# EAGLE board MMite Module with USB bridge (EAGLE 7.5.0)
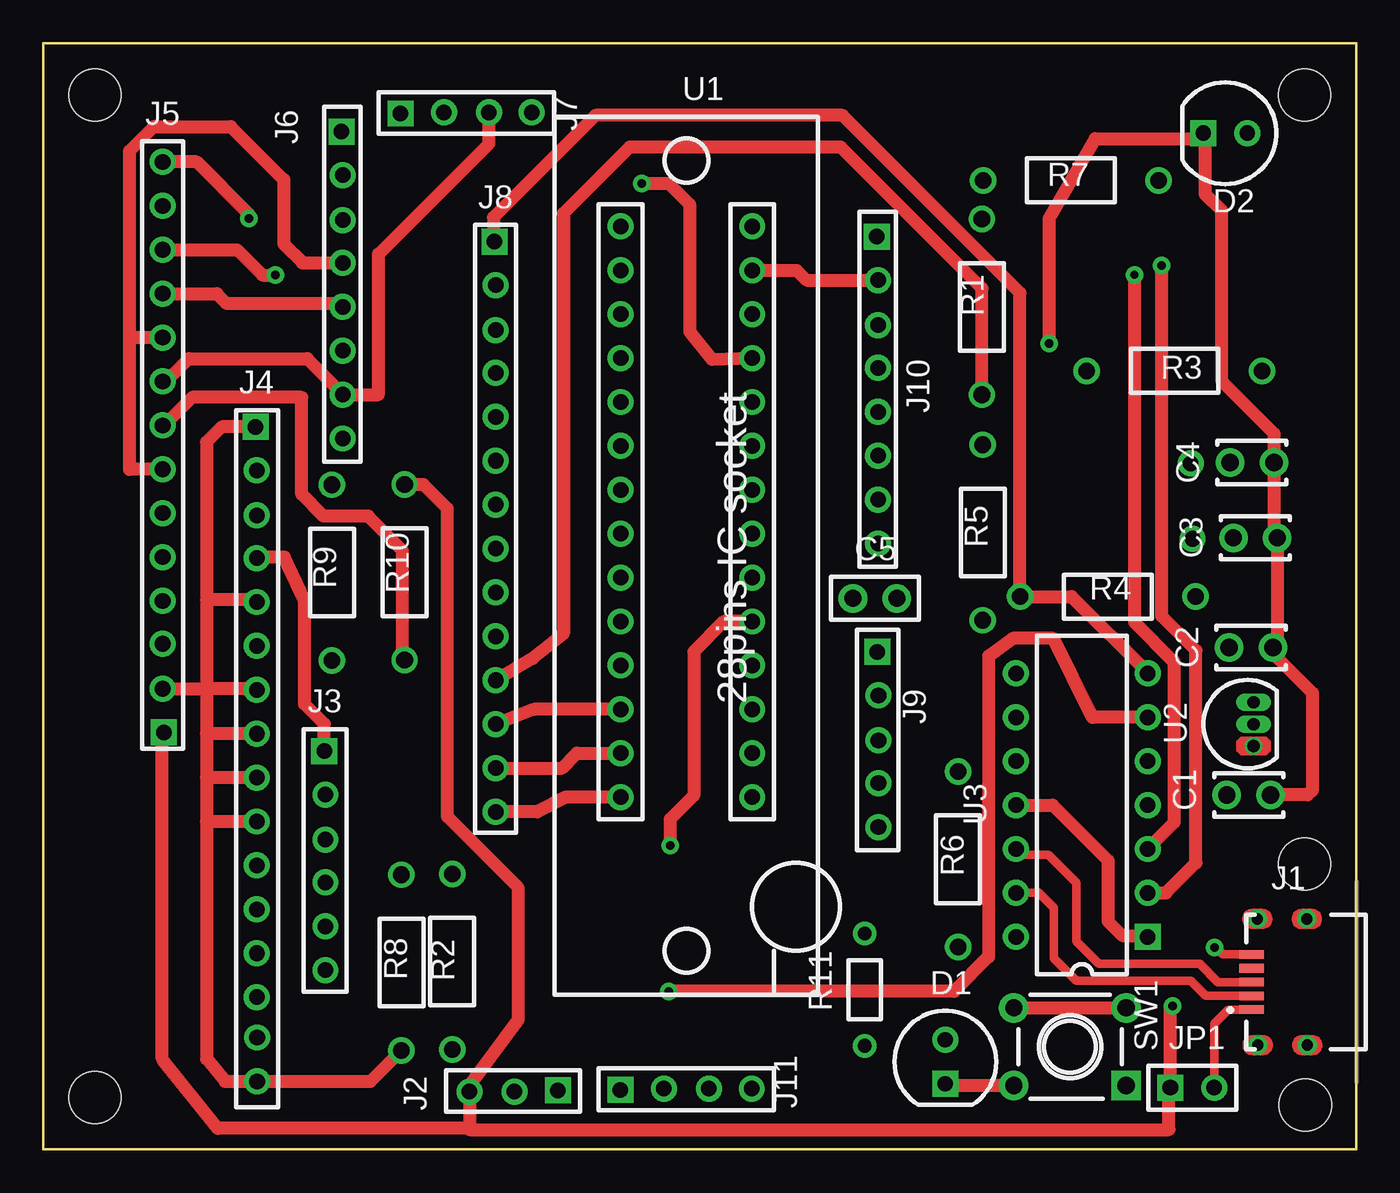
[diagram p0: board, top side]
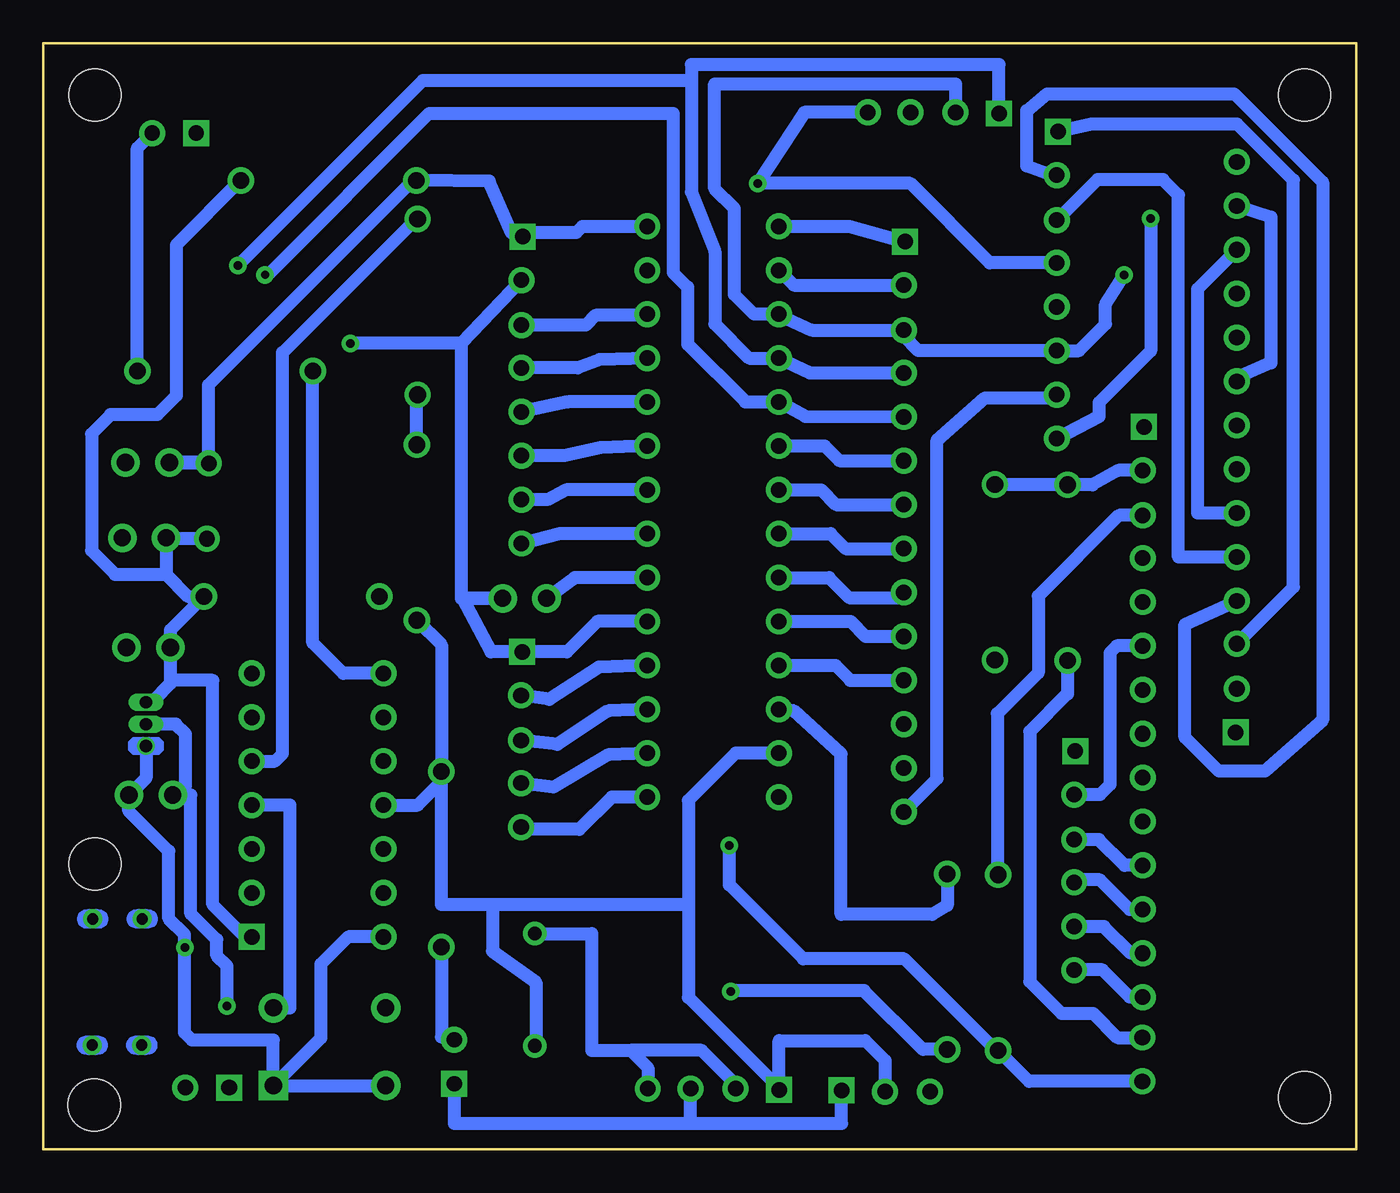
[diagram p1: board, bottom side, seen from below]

Size 76 x 64 mm. Coordinates in mm from the lower left corner, seen from the top.
Outline: 0,64 76,64 76,0 0,0 0,64
Copper layers (1*16): Top 0.035mm / dielectric 1.5mm / Bottom 0.035mm
Design rules "default *": minimum track width 10mil, minimum drill 0.61mm, track to track 8mil, track to pad 8mil, pad to pad 8mil, via to via 8mil, smd to smd 8mil, copper to edge 40mil, drill to drill 8mil, minimum pad ring 0mil, minimum via ring 8mil, stop-mask expansion 4mil, vias tented up to drill 19mil, thermal gap 10mil
Net classes: 0 Default: width 0.5 mm, clearance 0.33 mm
Holes 3 mm at 73.05,2.58 3,3 3,61 73,61 73,16.5

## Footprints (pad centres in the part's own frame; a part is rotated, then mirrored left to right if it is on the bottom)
CAP-2.54/4x2.5 = drill 1 pad 1.65: 1 -1.27,0; 2 1.27,0
CAP-2.54/5.1x2.5 = drill 1 pad 1.65: 1 -1.27,0; 2 1.27,0
LED-5Cil_Red = drill 0.889 pad 1.5 square: 1 -1.27,0 | drill 0.889 pad 1.5: 2 1.27,0
LED-5Cil_Green = drill 0.889 pad 1.5 square: 1 -1.27,0 | drill 0.889 pad 1.5: 2 1.27,0
Mini_USB_51387-578 = smd 0.5 x 1.4: 1 -1.6,1.75; 2 -0.8,1.75; 3 0,1.75; 4 0.8,1.75; 5 1.6,1.75 | drill 0.65 pad 1.1: 6 -3.65,1.396; 7 3.648,1.421; 8 -3.65,-1.472; 9 3.647,-1.447
CON3F = drill 0.9 pad 1.5 square: 1 -0.033,2.561 | drill 0.9 pad 1.5: 2 0.033,0.043; 3 0.033,-2.561
CON6F = drill 0.9 pad 1.5 square: 1 -0.033,6.339 | drill 0.9 pad 1.5: 2 0.033,3.821; 3 0.033,1.217; 4 0.033,-1.259; 5 0.033,-3.799; 6 0.033,-6.339
CON16F = drill 0.9 pad 1.5 square: 1 -0.044,18.937 | drill 0.9 pad 1.5: 2 0.022,16.419; 3 0.022,13.815; 4 0.022,11.339; 5 0.022,8.799; 6 0.022,6.259; 7 0.022,3.719; 8 0.022,1.179; 9 0.022,-1.361; 10 0.022,-3.901; 11 0.022,-6.441; 12 0.022,-8.981; 13 0.022,-11.521; 14 0.022,-14.061; 15 0.044,-16.397; 16 0.044,-18.937
CON14F = drill 0.9 pad 1.5 square: 1 -0.033,16.499 | drill 0.9 pad 1.5: 2 0.033,13.981; 3 0.033,11.377; 4 0.033,8.901; 5 0.033,6.361; 6 0.033,3.821; 7 0.033,1.281; 8 0.033,-1.259; 9 0.033,-3.799; 10 0.033,-6.339; 11 0.033,-8.879; 12 0.033,-11.419; 13 0.033,-13.959; 14 0.033,-16.499
CON8F = drill 0.9 pad 1.5 square: 1 -0.033,8.879 | drill 0.9 pad 1.5: 2 0.033,6.361; 3 0.033,3.757; 4 0.033,1.281; 5 0.033,-1.259; 6 0.033,-3.799; 7 0.033,-6.339; 8 0.033,-8.879
CON4F = drill 0.9 pad 1.5 square: 1 -0.033,3.799 | drill 0.9 pad 1.5: 2 0.033,1.281; 3 0.033,-1.323; 4 0.033,-3.799
CON5F = drill 0.9 pad 1.5 square: 1 -0.033,5.069 | drill 0.9 pad 1.5: 2 0.033,2.551; 3 0.033,-0.053; 4 0.033,-2.529; 5 0.033,-5.069
HDR-1x2 = drill 0.9 pad 1.5 square: 1 -1.27,0 | drill 0.9 pad 1.5: 2 1.27,0
Pad = drill 0.9 pad 1.5: 1 0,0
RES-10.16/5.1x2.5 = drill 0.965 pad 1.524: 1 -5.08,0; 2 5.08,0
RES-10.16/5.1x2.5_R3 = drill 0.965 pad 1.524: 1 -5.08,0; 2 5.08,0
RES-6.5/3.4x1.9 = drill 0.8 pad 1.35: 1 -3.25,0; 2 3.25,0
B3F-1 = drill 1 pad 1.7 square: 1 -3.25,2.25 | drill 1 pad 1.7: 2 3.25,2.25; 3 -3.25,-2.25; 4 3.25,-2.25
28pins_ZIF_pattern = drill 0.9 pad 1.5: 1 -3.81,17.78; 2 -3.81,15.24; 3 -3.81,12.7; 4 -3.81,10.16; 5 -3.81,7.62; 6 -3.81,5.08; 7 -3.81,2.54; 8 -3.81,0; 9 -3.81,-2.54; 10 -3.81,-5.08; 11 -3.81,-7.62; 12 -3.81,-10.16; 13 -3.81,-12.7; 14 -3.81,-15.24; 15 3.81,-15.24; 16 3.81,-12.7; 17 3.81,-10.16; 18 3.81,-7.62; 19 3.81,-5.08; 20 3.81,-2.54; 21 3.81,0; 22 3.81,2.54; 23 3.81,5.08; 24 3.81,7.62; 25 3.81,10.16; 26 3.81,12.7; 27 3.81,15.24; 28 3.81,17.78
TO-92 = drill 0.7 pad 1: 1 -1.27,0 | drill 0.7 pad 1 long: 2 0,0; 3 1.27,0
DIP-14 = drill 0.9 pad 1.5 square: 1 -3.81,7.62 | drill 0.9 pad 1.5: 2 -3.81,5.08; 3 -3.81,2.54; 4 -3.81,0; 5 -3.81,-2.54; 6 -3.81,-5.08; 7 -3.81,-7.62; 8 3.81,-7.62; 9 3.81,-5.08; 10 3.81,-2.54; 11 3.81,0; 12 3.81,2.54; 13 3.81,5.08; 14 3.81,7.62

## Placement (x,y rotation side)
C1  10uF  [CAP-2.54/4x2.5]  69.77,20.51 0 top
C2  10uF  [CAP-2.54/4x2.5]  69.91,29.04 0 top
C3  100nF  [CAP-2.54/4x2.5]  70.15,35.39 0 top
C4  100nF  [CAP-2.54/4x2.5]  69.96,39.74 0 top
C5  47uF-16V Tan  [CAP-2.54/5.1x2.5]  48.14,31.88 0 top
D1  RED  [LED-5Cil_Red]  52.21,5.07 90 top
D2  GREEN  [LED-5Cil_Green]  68.42,58.79 0 top
J1  MINI USB  [Mini_USB_51387-578]  71.69,9.68 90 top
J2  POWER I/O  [CON3F]  27.23,3.38 270 top
J3  LCD 16X2  [CON6F]  16.3,16.71 0 top
J4  CON16F  [CON16F]  12.34,22.87 0 top
J5  CON14F  [CON14F]  6.95,40.63 180 top
J6  LCD ILI9341  [CON8F]  17.3,50.01 0 top
J7  ILI9341-SD  [CON4F]  24.48,59.96 90 top
J8  MM I/O  [CON14F]  26.15,36.02 0 top
J9  MM I/O  [CON5F]  48.31,23.71 0 top
J10  MM I/O  [CON8F]  48.28,43.93 0 top
J11  UNI/O-TEMP  [CON4F]  37.21,3.48 90 top
JP1  JUMPER  [HDR-1x2]  66.51,3.58 0 top
Pad1  PAD  [Pad]  66.41,39.69 0 top
Pad2  PAD  [Pad]  66.53,35.33 0 top
R1  1K5  [RES-10.16/5.1x2.5]  54.33,48.74 270 top
R2  1K5  [RES-10.16/5.1x2.5]  23.67,10.86 90 top
R3  1K  [RES-10.16/5.1x2.5_R3]  65.47,45.04 0 top
R4  10K  [RES-10.16/5.1x2.5_R3]  61.62,31.98 180 top
R5  10K  [RES-10.16/5.1x2.5]  54.38,35.69 90 top
R6  1K5  [RES-10.16/5.1x2.5]  52.95,16.78 270 top
R7  10R  [RES-10.16/5.1x2.5_R3]  59.48,56.06 180 top
R8  1K8  [RES-10.16/5.1x2.5]  20.74,10.81 270 top
R9  1K8  [RES-10.16/5.1x2.5]  16.71,33.37 270 top
R10  18R  [RES-10.16/5.1x2.5]  20.92,33.39 270 top
R11  100K  [RES-6.5/3.4x1.9]  47.55,9.24 90 top
SW1  SWITCH_2DIP  [B3F-1]  59.43,5.94 180 top
U1  28PINS_ZIF_SOCKET  [28pins_ZIF_pattern]  37.23,35.62 0 top
U2  MCP1700-33  [TO-92]  70.05,24.61 90 top
U3  PIC16F1455  [DIP-14]  60.11,19.92 180 top

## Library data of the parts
C1-C4 = common; DESCRIPTION: Non-polarized
C5 = common; ATTR_1: Electrolytic; DESCRIPTION: Polarized
D1 D2 = common; DESCRIPTION: LED
J1 J2 J7 J11 = common; DATASHEET: http://datasheets.diptrace.com/con_board_in/510221400_sd.pdf; MANUFACTURER: Molex
J3 J5 J8-J10 JP1 Pad1 Pad2 = common
J4 = common; DATASHEET: http://datasheets.diptrace.com/con_board_in/DF4.pdf; MANUFACTURER: Hirose
J6 = common; DATASHEET: http://datasheets.diptrace.com/con_board_in/510150300_sd.pdf; MANUFACTURER: Molex
R1-R11 = common; DESCRIPTION: Fixed Resistor
SW1 = common; ATTR_1: 2 Positions; DESCRIPTION: DIP Switch
U1 = common; MANUFACTURER: MICROMITE
U2 = common; DATASHEET: http://datasheets.diptrace.com/microchip/22008d.pdf; MANUFACTURER: Microchip
U3 = common; DATASHEET: http://datasheets.diptrace.com/microchip/21203Q.pdf; MANUFACTURER: Microchip

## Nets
Net_0: J8.1 R4.2 U1.1 U3.7
Net_1: C1.2 C2.2 C3.2 C4.2 C5.2 D1.1 D2.1 J1.5 J2.1 J4.1 J4.5 J4.7 J4.8 J4.9 J4.10 J4.16 J5.2 J9.1 J10.2 J11.3 R8.2 SW1.1 SW1.2 U1.19 U1.27 U2.1 U3.14
Net_2: C2.1 C3.1 J2.2 J8.13 J11.1 Pad2.1 R4.1 R5.1 R6.1 R7.1 R11.1 U1.13 U2.3 U3.1 U3.11
Net_3: J7.1 J8.4 U1.4 U3.2
Net_4: J8.5 U1.5 U3.3
Net_5: SW1.3 SW1.4 U3.4
Net_6: R1.1 U3.5
Net_7: J8.11 R1.2 R5.2 U1.11
Net_8: R2.1 U3.6
Net_9: J8.12 R2.2 U1.12
Net_10: R3.1 U3.8
Net_11: J1.3 U3.12
Net_12: D2.2 R3.2
Net_13: J1.2 U3.13
Net_14: C1.1 J1.1 J2.3 J4.2 J5.1 JP1.1 JP1.2 R9.1 R10.1 U2.2
Net_15: C5.1 U1.20
Net_16: D1.2 R6.2
Net_17: C4.1 J10.1 Pad1.1 R7.2 U1.28
Net_18: J3.1 J4.4
Net_19: J4.3 R8.1
Net_20: J11.2 J11.4 R11.2
Net_21: J3.6 J4.14
Net_22: J3.5 J4.13
Net_23: J3.4 J4.12
Net_24: J3.3 J4.11
Net_25: J3.2 J4.6
Net_26: J4.15 R9.2
Net_27: J9.2 U1.18
Net_28: J9.3 U1.17
Net_29: J9.4 U1.16
Net_30: J9.5 U1.15
Net_31: J10.3 U1.26
Net_32: J5.7 J5.10 J6.4 J7.4 J10.4 U1.25
Net_33: J10.5 U1.24
Net_34: J10.6 U1.23
Net_35: J10.7 U1.22
Net_36: J10.8 U1.21
Net_37: J8.2 U1.2
Net_38: J5.6 J5.12 J6.6 J7.2 J8.3 U1.3
Net_39: J8.6 U1.6
Net_40: J8.7 U1.7
Net_41: J8.8 U1.8
Net_42: J8.9 U1.9
Net_43: J8.10 U1.10
Net_44: J5.9 J5.13 J6.7 J7.3 J8.14 U1.14
Net_45: J5.8 R10.2
Net_49: J5.14 J6.8
Net_50: J5.11 J6.5
Net_51: J5.5 J6.3
Net_52: J5.4 J6.2
Net_53: J5.3 J6.1

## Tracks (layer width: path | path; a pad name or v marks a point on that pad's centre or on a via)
Net_0
  Top 0.75: J8.1 26.06,52.42 26.06,53.92 31.97,59.83 46.26,59.83 56.54,49.55 R4.2 59.52,31.98 63.92,27.58 U3.7
  Bottom 0.75: U1.1 29.33,53.4 J8.1
Net_1  (via drill 0.49 pad 1.02)
  Top 0.5: J1.5 68.28,11.28 67.89,11.67 v67.79,11.67
  Top 0.75: SW1.2 52.21,3.69 D1.1 | v58.22,46.64 58.22,53.87 60.89,58.48 66.83,58.48 D2.1 67.24,58.8 67.24,55.27 68.19,54.33 68.19,44.47 71.23,41.43 C4.2 71.23,35.58 C3.2 71.42,29.28 C2.2 71.18,28.69 73.45,26.42 73.45,20.79 73.17,20.51 C1.2 | U1.27 43.61,50.86 44.18,50.29 J10.2 | U1.19 39.41,30.54 37.65,28.79 37.65,20.48 36.28,19.11 v36.28,17.57 | J4.1 10.33,41.81 9.46,40.93 9.46,31.8 | 9.46,31.8 9.46,26.65 | 9.46,26.65 9.46,24.05 | 9.46,24.05 9.46,21.51 | 9.46,21.51 9.46,18.97 | 9.46,18.97 9.46,5.23 10.53,3.93 J4.16 18.94,3.93 R8.2 | J4.5 12.36,31.8 9.46,31.8 | J4.7 12.36,26.65 9.46,26.65 | J4.8 9.46,24.05 | J4.9 9.46,21.51 | J4.10 9.46,18.97 | J5.2 9.46,26.65
  Bottom 0.75: SW1.1 SW1.2 | SW1.2 | J10.2 51.8,46.64 | 51.8,46.64 v58.22,46.64 | 51.8,46.64 51.8,31.88 C5.2 51.73,31.88 50.09,28.78 J9.1 45.68,28.78 43.92,30.54 U1.19 | SW1.1 62.68,6.33 67.38,6.33 67.82,6.76 67.82,11.63 | 67.82,11.63 67.82,12.45 68.72,13.35 68.72,17.26 71.04,19.57 C1.2 70.05,21.5 U2.1 | D1.1 52.21,1.5 38.55,1.5 | 38.55,1.5 29.79,1.5 J2.1 | J11.3 38.55,3.51 38.55,1.5 | v67.79,11.67 67.82,11.63 | U3.14 58.35,12.3 59.93,10.72 59.93,6.43 SW1.1 | v36.28,17.57 36.28,15.3 32.01,11.02 26.16,11.02 20.86,5.73 R8.2 18.94,3.93 J4.16
Net_2
  Top 0.75: J8.13 30.02,22.06 30.88,22.92 U1.13 | U3.11 58.43,19.92 61.63,16.72 61.63,13.2 62.47,12.37 63.86,12.37 U3.1
  Bottom 0.75: 68.88,33.27 C3.1 68.83,35.33 Pad2.1 | 68.88,33.27 67.6,31.98 R4.1 68.64,30.04 C2.1 68.64,26.94 69.7,25.88 | R5.1 52.95,29.19 R6.1 | R7.1 68.3,52.32 68.3,43.6 69.39,42.51 72.1,42.51 73.2,41.4 73.2,34.64 71.83,33.27 68.88,33.27 | J2.2 27.27,5.15 28.41,6.3 33.41,6.3 J11.1 33.41,3.56 38.65,8.8 38.65,14.16 | U1.13 35.92,22.92 38.65,20.19 38.65,14.16 | 38.65,14.16 49.99,14.16 | 49.99,14.16 49.99,11.47 47.48,9.66 47.48,5.99 R11.1 | U3.1 64.33,12.3 66.19,14.16 66.19,27.13 68.45,27.13 69.7,25.88 | 69.7,25.88 U2.3 69.7,25.88 | 49.99,14.16 52.95,14.16 R6.1 | U3.11 54.32,19.92 52.95,21.29 R6.1
Net_3  (via drill 0.49 pad 1.02)
  Top 0.75: U3.2 64.98,14.84 66.72,16.58 66.72,28.88 64.74,30.85 v64.74,51.13
  Bottom 0.75: J8.4 31.62,44.92 U1.4 35.15,45.78 37.12,47.76 37.12,51.95 38.48,55.38 38.48,61.86 | J7.1 20.68,62.76 38.48,62.76 38.48,61.86 | v64.74,51.13 54.02,61.86 38.48,61.86
Net_4  (via drill 0.49 pad 1.02)
  Top 0.75: v63.16,50.6 63.16,30.52 65.45,28.23 65.45,18.9 U3.3
  Bottom 0.75: J8.5 31.89,42.41 U1.5 35.37,43.24 38.7,46.58 38.7,49.88 39.54,50.72 39.54,59.95 53.66,59.95 63.11,50.49 v63.16,50.6
Net_5
  Top 0.75: SW1.4 | SW1.4 SW1.3
  Bottom 0.75: SW1.3 61.72,8.19 61.72,19.92 U3.4
Net_6
  Bottom 0.75: U3.5 62.59,22.46 62.14,22.9 62.14,46.1 54.41,53.82 R1.1
Net_7
  Top 0.75: R1.2 54.33,49.82 46.17,57.98 33.95,57.98 30.11,54.15 30.11,29.84 28.33,28.4 J8.11
  Bottom 0.75: U1.11 30.14,28 29.28,27.14 J8.11 | R5.2 54.38,43.66 R1.2
Net_8  (via drill 0.49 pad 1.02)
  Top 0.75: U3.6 60.73,25 58.46,29.56 56.12,29.56 54.72,28.53 54.72,11.13 52.73,9.14 v36.2,9.14
  Bottom 0.75: R2.1 25.07,5.78 28.48,9.19 36.2,9.19 v36.2,9.14
Net_9
  Top 0.75: U1.12 28.39,25.46 J8.12
  Bottom 0.75: R2.2 23.67,14.12 24.55,13.6 29.82,13.6 29.82,22.88 32.56,25.37 U1.12
Net_10
  Bottom 0.75: U3.8 58.63,27.54 60.39,29.3 R3.1
Net_11
  Top 0.5: J1.3 68,9.68 66.95,10.73 61.11,10.73 59.8,12.03 59.8,15.41 58.16,17.06 56.63,17.06 U3.12
Net_12
  Bottom 0.75: R3.2 70.55,57.93 D2.2
Net_13
  Top 0.5: J1.2 67.3,8.88 66.42,9.77 59.8,9.77 58.5,11.07 58.5,13.97 57.63,14.84 U3.13
Net_14  (via drill 0.49 pad 1.02)
  Top 0.5: JP1.2 67.78,7.27 68.59,8.08 J1.1
  Top 0.75: J2.3 | J2.3 24.67,1.22 | 24.67,1.22 10.1,1.22 6.89,5.23 6.89,23.68 J5.1 | R10.1 21.99,38.48 23.38,37.09 23.38,19.26 27.48,15.16 27.48,7.47 24.56,3.54 J2.3 | v65.36,8.3 65.23,8.17 JP1.1 65.16,3.5 65.16,1.14 24.67,1.14 24.67,1.22 | J2.3
  Bottom 0.75: 20.49,38.45 R10.1 | R10.1 | J4.2 13.79,39.29 15.27,38.45 R9.1 16.81,38.48 R10.1 | U2.2 68.33,24.61 67.76,24.04 67.76,21.02 68.5,20.28 C1.1 67.46,20.51 67.46,13.63 65.95,12.13 65.95,11.21 65.36,10.62 v65.36,8.3
Net_15
  Bottom 0.75: U1.20 45.24,33.08 47.11,31.7 C5.1
Net_16
  Bottom 0.75: R6.2 52.95,6.5 52.21,6.5 D1.2
Net_17
  Bottom 0.75: J10.1 48.67,52.81 48.9,53.05 | 48.9,53.05 50.18,56.03 R7.2 54.4,56.27 66.45,44.22 66.45,39.75 C4.1 68.64,39.69 Pad1.1 | U1.28 44.8,53.39 45.15,53.05 48.9,53.05
Net_18
  Top 0.75: J3.1 16.27,24.62 15.13,25.76 15.13,31.73 13.95,34.27 12.36,34.27 J4.4
Net_19
  Bottom 0.75: J4.3 13.74,36.69 18.41,32.01 18.41,27.57 20.78,25.21 20.78,15.93 R8.1
Net_20
  Bottom 0.75: R11.2 44.26,12.49 44.26,5.73 42.02,5.73 | 42.02,5.73 41.01,4.72 J11.4 | J11.2 35.93,3.76 37.89,5.73 42.02,5.73
Net_21
  Bottom 0.75: J4.14 13.12,8.81 14.7,10.38 16.32,10.38 J3.6
Net_22
  Bottom 0.75: J4.13 13.06,11.35 14.6,12.9 16.32,12.9 J3.5
Net_23
  Bottom 0.75: J4.12 13.12,13.89 14.83,15.6 16.18,15.6 J3.4
Net_24
  Bottom 0.75: J4.11 13.4,16.43 14.89,17.92 J3.3
Net_25
  Bottom 0.75: J4.6 13.86,29.13 14.26,28.73 14.26,21.1 14.84,20.53 J3.2
Net_26
  Bottom 0.75: R9.2 16.71,26.35 18.9,24.17 18.9,9.71 17.06,7.87 15.23,7.87 13.83,6.47 J4.15
Net_27
  Bottom 0.75: U1.18 43.83,27.91 46.7,26.04 J9.2
Net_28
  Bottom 0.75: U1.17 43.3,25.37 46.23,23.43 J9.3
Net_29
  Bottom 0.75: U1.16 43.31,22.83 46.47,20.96 J9.4
Net_30
  Bottom 0.75: U1.15 43.1,20.38 44.97,18.51 48.21,18.51 J9.5
Net_31
  Bottom 0.75: U1.26 41.23,48.25 44.03,48.25 44.59,47.69 J10.3
Net_32  (via drill 0.49 pad 1.02)
  Top 0.75: U1.25 38.73,45.69 37.43,47.31 37.43,54.66 36.21,55.88 v34.65,55.88 | J5.10 5,46.97 | 5,46.97 5,57.77 6.41,59.18 10.86,59.18 13.93,56.11 13.93,52.37 15.01,51.29 J6.4 | J5.7 5,39.35 5,46.97
  Bottom 0.75: U1.25 43.8,45.69 45.05,45.21 J10.4 | J6.4 21.22,51.29 25.82,55.88 v34.65,55.88 31.95,60 J7.4
Net_33
  Bottom 0.75: U1.24 45.64,43.24 J10.5
Net_34
  Bottom 0.75: U1.23 43.75,40.61 45.82,40.13 J10.6
Net_35
  Bottom 0.75: U1.22 45.74,38.16 46.81,37.59 J10.7
Net_36
  Bottom 0.75: U1.21 46.09,35.62 J10.8
Net_37
  Bottom 0.75: U1.2 32.56,50 J8.2
Net_38  (via drill 0.49 pad 1.02)
  Top 0.75: J5.12 11.22,52.05 12.69,50.58 v13.44,50.58
  Bottom 0.75: J7.2 23.2,61.64 37.13,61.64 37.13,55.59 35.99,54.45 35.99,49.46 34.86,48.32 U1.3 33.34,48.25 31.52,47.4 J8.3 26.19,47.03 25.36,46.21 J6.6 16.06,46.21 14.52,47.75 14.52,48.89 13.4,50.66 v13.44,50.58 | J5.6 9.18,36.81 9.18,49.78 J5.12
Net_39
  Bottom 0.75: U1.6 30.77,40.7 29.91,39.84 J8.6
Net_40
  Bottom 0.75: U1.7 30.97,38.16 30.11,37.3 J8.7
Net_41
  Bottom 0.75: U1.8 30.42,35.62 29.56,34.76 J8.8
Net_42
  Bottom 0.75: U1.9 30.52,33.08 29.35,31.92 26.49,31.92 J8.9
Net_43
  Bottom 0.75: U1.10 29.26,30.54 28.4,29.68 J8.10
Net_44
  Top 0.75: U1.14 30.24,20.38 28.59,19.52 J8.14 | J7.3 25.8,58.19 19.4,51.79 19.4,43.67 J6.7 17.33,43.7 15.28,45.75 8.43,45.75 7.12,44.43 J5.9
  Bottom 0.75: J8.14 24.26,21.45 24.26,41.04 21.48,43.48 17.33,43.48 J6.7 | J5.13 4.95,53.95 4.95,45.51 6.66,44.77 J5.9
Net_45
  Top 0.75: R10.2 | R10.2 20.8,28.54 20.8,34.64 18.81,36.63 16.22,36.63 14.96,37.89 14.96,43.51 8.63,43.51 7,41.89 J5.8
Net_49  (via drill 0.49 pad 1.02)
  Top 0.75: v11.9,53.87 11.9,54.1 8.87,57.13 J5.14
  Bottom 0.75: v11.9,53.87 11.9,46.2 14.89,43.21 14.89,42.4 J6.8
Net_50
  Top 0.75: J5.11 10.04,49.51 10.59,48.96 17.12,48.96 J6.5
Net_51
  Bottom 0.75: J5.5 10.29,34.27 10.29,55.22 11.19,56.11 14.98,56.11 J6.3
Net_52
  Bottom 0.75: J6.2 17.65,56.37 19.08,56.89 19.08,60.09 17.9,61.08 7.06,61.08 1.95,55.96 1.95,24.83 5.29,21.88 7.96,21.88 9.91,23.84 9.91,30.38 J5.4
Net_53
  Bottom 0.75: J5.3 3.64,32.53 3.64,56.07 6.89,59.32 15.34,59.32 J6.1

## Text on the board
tDocu: SD | CS | CS | MO | MI | RESET | SCK | 1 | 1 | D/C | T-CLK(25) | 28 | T-CS | T-DIN(3) | T-DO(14) | 1 | T-IRQ | 21 | LCD ILI9341 MODULE | 1 | 19 | 14 | RS | EN | 15 | D4 | +5 | D5 | D6 | D7 | POWER I/O | EEPROM | /TEMP | LCD 16X2 MODULE | +5 | +3.3 | GND | +3.3 | I/O | GND | MM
